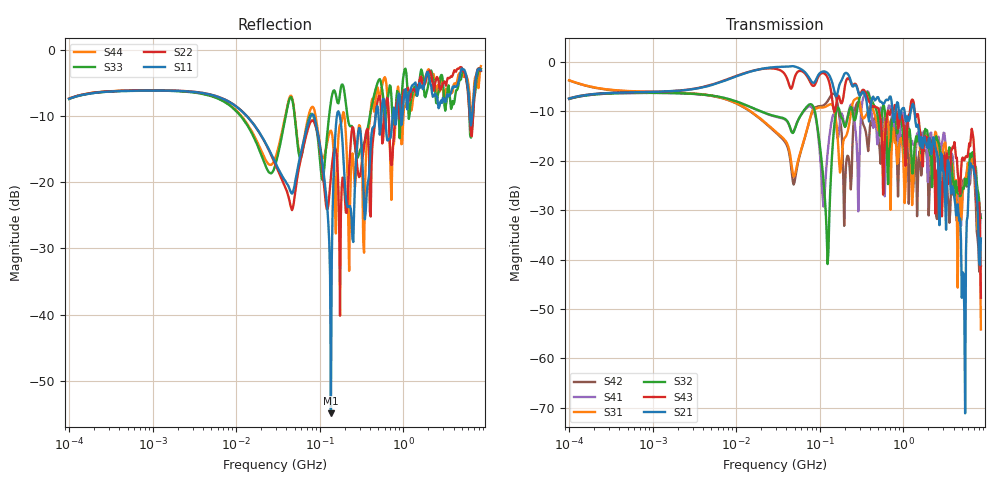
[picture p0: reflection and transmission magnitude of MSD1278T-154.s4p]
# MHz S MA R 50
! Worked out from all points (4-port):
!   498 points, 100 kHz to 8.5 GHz, reference 50 ohm
!   strongest paths, dB at 100 kHz, 1.698 MHz, 29.49 MHz, 500.7 MHz, 8.5 GHz:
!     S21: -7.4, -5.9, -1.0, -7.1, -35.7
!     S43: -7.4, -5.9, -1.3, -9.3, -47.7
!     S32: -7.5, -6.3, -10.9, -11.5, -31.6
!     S31: -3.7, -6.1, -14.0, -13.8, -54.2
!     S41: -7.5, -6.3, -11.0, -16.2, -30.8
!     S42: -3.7, -6.2, -14.2, -15.2, -41.4
!   lowest |S11| = -54.9 dB at 136.2 MHz (marker M1), VSWR 1.00, Z = 49.9 - j0.117 ohm
!   |S11| at or under -10 dB: 174.1 MHz to 467.1 MHz (293 MHz wide, 91.4 % of centre); 609.3 MHz to 747.5 MHz (138.3 MHz wide, 20.4 % of centre); 6.292 GHz to 6.669 GHz (376.3 MHz wide, 5.81 % of centre)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
0.1  0.427 28.3  0.4279 29.6  0.6548 -18.9  0.4238 -151.5
     0.4279 29.6  0.4283 28.4  0.4238 -151.4  0.6532 -19.1
     0.6548 -18.9  0.4238 -151.4  0.4257 28.5  0.4286 29.5
     0.4238 -151.5  0.6532 -19.1  0.4286 29.5  0.4288 28.6
136.2065  0.001792 -139.1  0.6784 -46.8  0.3757 6.3  0.2297 58.2
          0.6784 -46.8  0.11 0.7  0.06986 121.3  0.4575 23.7
          0.3757 6.3  0.06986 121.3  0.405 13.6  0.5174 -63.7
          0.2297 58.2  0.4575 23.7  0.5174 -63.7  0.2455 -41.3
167.2873  0.3437 -9.1  0.5348 -23.9  0.1325 -109.6  0.1754 29.2
          0.5348 -23.9  0.08968 -90.2  0.3458 44.2  0.3279 -49.5
          0.1325 -109.6  0.3458 44.2  0.3944 -28.7  0.4583 -33.1
          0.1754 29.2  0.3279 -49.5  0.4583 -33.1  0.218 31.7
2365.873  0.4572 169.6  0.1533 61.0  0.1715 141.0  0.1036 114.7
          0.1533 61.0  0.5199 175.9  0.1474 138.8  0.09458 80.4
          0.1715 141.0  0.1474 138.8  0.5639 154.4  0.1023 41.3
          0.1036 114.7  0.09458 80.4  0.1023 41.3  0.602 153.0
5261.791  0.7132 -101.5  0.00718 68.9  0.05482 -114.1  0.05755 -110.0
          0.00718 68.9  0.6873 -107.9  0.05192 -132.8  0.06477 -130.7
          0.05482 -114.1  0.05192 -132.8  0.6965 -101.2  0.102 153.1
          0.05755 -110.0  0.06477 -130.7  0.102 153.1  0.6255 -101.8
6764.496  0.3495 49.2  0.08876 26.8  0.09867 32.1  0.1201 68.5
          0.08876 26.8  0.2718 66.6  0.1226 49.9  0.09174 38.0
          0.09867 32.1  0.1226 49.9  0.2843 51.2  0.1908 -35.9
          0.1201 68.5  0.09174 38.0  0.1908 -35.9  0.3458 68.2
8500  0.7023 -56.2  0.01637 -25.6  0.00196 -145.6  0.02878 -109.6
      0.01637 -25.6  0.6918 -57.4  0.02641 171.4  0.008525 -131.2
      0.00196 -145.6  0.02641 171.4  0.7195 -49.7  0.004112 -121.7
      0.02878 -109.6  0.008525 -131.2  0.004112 -121.7  0.7534 -48.9
